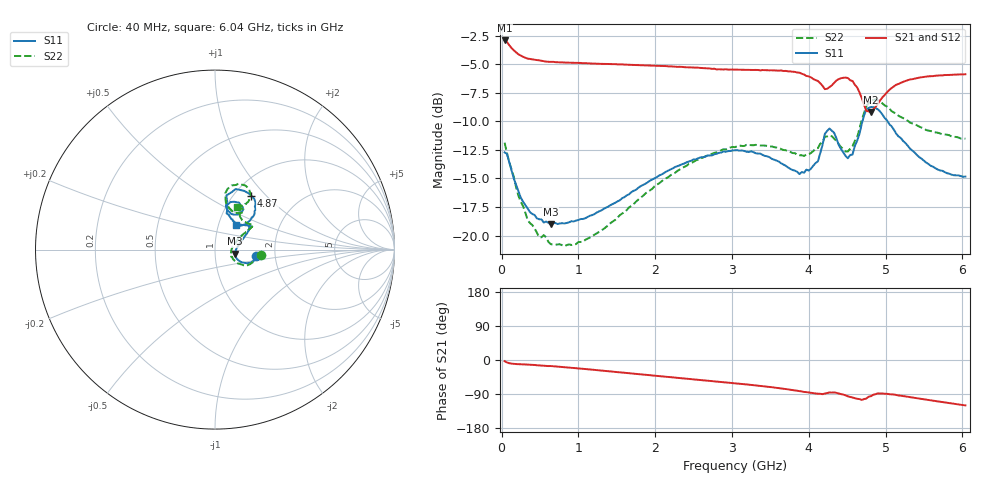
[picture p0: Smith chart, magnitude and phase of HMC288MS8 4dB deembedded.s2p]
!Hittite Microwave Corporation
!12 Elizabeth Drive
!Chelmsford, MA 01824
!Tel: 978-250-3343
!Fax: 978-250-3373
!Device: HMC288MS8, 0.7-3.7 GHz GaAs IC 3-bit Digital Attenuator in 8-lead Grounded Base surface Mount Plastic Package
!Misc:  4dB state, room
# GHZ S DB R 50.0
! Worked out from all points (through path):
!   201 points, 40 MHz to 6.04 GHz, reference 50 ohm
!   highest |S21| = -2.91 dB at 40 MHz (marker M1); lowest = -9.2 dB at 4.81 GHz (marker M2)
!   group delay of S21, straight-line fit = 51.7 ps
!   lowest |S11| = -19.0 dB at 640 MHz (marker M3), VSWR 1.25, Z = 62.2 - j2.93 ohm
!   |S11| at or under -10 dB: start of sweep to 4.7 GHz; 5.027 GHz to end of sweep
!   |S22| runs from -20.9 to -8.1 dB; largest |S21 - S12| = 0.005
!   S11 on the Smith chart (normalised r, x): 40 MHz: 1.59, -0.12; 4.87 GHz: 1.20, +0.83; 6.04 GHz: 1.21, +0.35
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0.04  -12.72 -8.7  -2.91 -3.2  -2.86 -3.0  -11.87 -6.4
0.13  -14.28 -23.1  -3.57 -9.5  -3.54 -9.4  -14.20 -27.6
0.34  -17.63 -22.7  -4.50 -12.1  -4.46 -12.0  -18.63 -28.3
0.64  -19.03 -12.0  -4.79 -15.9  -4.78 -16.2  -20.75 -14.7
1.06  -18.55 1.7  -4.91 -23.3  -4.90 -23.4  -20.55 4.0
2.05  -14.75 24.3  -5.14 -42.4  -5.12 -42.5  -15.44 27.9
3.04  -12.54 34.0  -5.46 -61.5  -5.45 -61.6  -12.26 31.8
3.37  -12.83 36.5  -5.53 -68.3  -5.49 -68.5  -12.12 33.3
3.88  -14.62 52.9  -5.74 -82.2  -5.72 -82.3  -12.97 44.0
4.06  -13.88 66.3  -6.29 -87.3  -6.27 -87.6  -12.61 54.2
4.18  -12.06 75.7  -6.89 -90.2  -6.87 -90.5  -11.83 58.6
4.27  -10.63 62.9  -7.00 -85.6  -7.00 -85.9  -11.22 54.5
4.36  -11.47 54.5  -6.42 -86.6  -6.40 -86.7  -11.74 53.3
4.51  -13.23 65.5  -6.20 -95.8  -6.19 -95.8  -12.64 64.8
4.57  -12.91 71.3  -6.46 -99.1  -6.47 -99.1  -12.19 71.5
4.69  -10.24 78.2  -7.95 -105.3  -7.94 -105.3  -9.90 79.6
4.75  -8.96 71.2  -9.08 -101.7  -9.04 -101.2  -8.66 75.6
4.81  -8.74 63.5  -9.19 -95.5  -9.18 -95.7  -8.17 70.4
4.87  -8.83 56.0  -8.74 -90.1  -8.84 -90.2  -8.07 64.9
5.05  -10.25 44.1  -7.24 -90.2  -7.22 -90.0  -8.86 56.3
5.53  -13.62 41.4  -6.08 -104.6  -6.06 -104.8  -10.76 57.4
6.04  -14.84 50.0  -5.87 -119.8  -5.88 -120.0  -11.52 62.2
